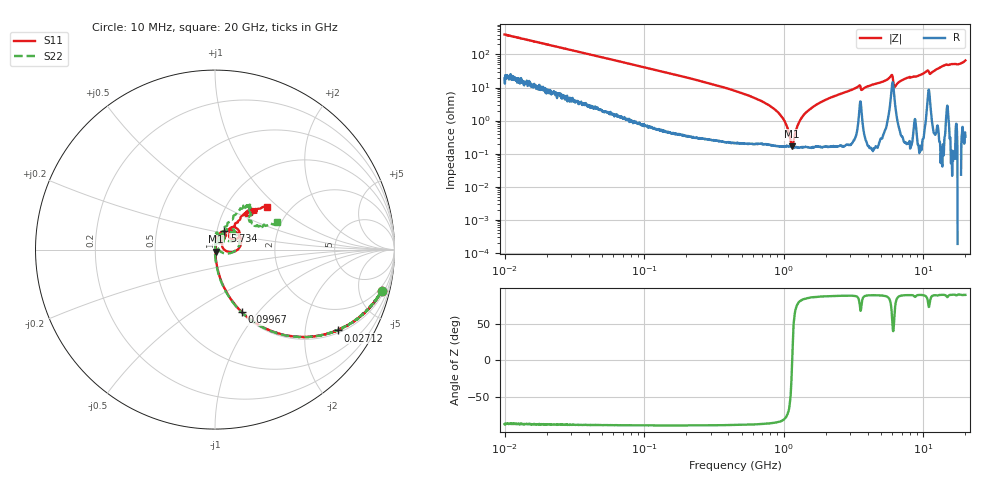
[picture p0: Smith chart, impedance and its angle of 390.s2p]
!Keysight Technologies,P5008B,MY61100088,A.16.20.02
!Date: Friday, August 30, 2024 14:09:02
!Correction: S11(C  2-Port  )
!S21(C  2-Port  )
!S12(C  2-Port  )
!S22(C  2-Port  )
!S2P File: Measurements: S11, S21, S12, S22:Log Frequency Sweep
# Hz S  MA  R 50
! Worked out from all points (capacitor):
!   1601 points, 10 MHz to 20 GHz, reference 50 ohm
!   read as one part in series: C = 39.7 pF near 10.39 MHz
!   lowest |Z| = 165 mohm at 1.146 GHz (marker M1)
!   series resonance near 1.147 GHz, so ESL is about 480 pH
!   S11 on the Smith chart (normalised r, x): 10 MHz: 1.36, -8.01; 27.12 MHz: 1.09, -2.97; 99.67 MHz: 1.01, -0.83; 5.734 GHz: 1.09, +0.23; 20 GHz: 1.53, +0.85
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1e7  0.9602 -13.8  0.2395 73.5  0.2395 73.5  0.9597 -13.9
2.711816e7  0.8189 -33.4  0.5504 54.9  0.5502 54.9  0.8188 -33.5
3.555162e7  0.7423 -40.4  0.6483 47.8  0.6482 47.8  0.7422 -40.5
9.966934e7  0.3793 -66.8  0.9191 22.1  0.9189 22.1  0.3794 -67.0
1.263918e8  0.3084 -71.2  0.9466 17.8  0.9462 17.8  0.3085 -71.4
4.472136e8  0.08415 -83.5  0.9945 4.2  0.9942 4.2  0.08405 -85.1
8.452326e8  0.03253 -83.5  0.9978 0.8  0.9975 0.8  0.03234 -89.0
1.145559e9  0.01272 -70.7  0.9984 -0.7  0.9982 -0.7  0.01214 -95.5
1.253768e9  0.007074 -60.9  0.9986 -1.1  0.9982 -1.1  0.00637 -96.4
1.378733e9  0.002306 0.7  0.9987 -1.6  0.9983 -1.6  0.000948 7.0
1.589917e9  0.00793 67.0  0.9987 -2.4  0.9983 -2.4  0.00716 84.9
2.114282e9  0.02432 80.2  0.9984 -4.1  0.9981 -4.1  0.0239 83.0
5.652411e9  0.1072 68.5  0.9805 -15.3  0.9803 -15.4  0.1088 63.1
5.733545e9  0.1168 63.4  0.9719 -16.0  0.9717 -16.0  0.116 60.7
5.927413e9  0.1531 40.2  0.9083 -16.9  0.9078 -17.0  0.146 33.8
6.425969e9  0.04667 30.1  0.9881 -12.4  0.9875 -12.5  0.03163 81.2
7.697294e9  0.09098 56.6  0.9973 -17.7  0.9969 -17.8  0.08744 82.3
9.08967e9  0.07903 57.0  0.9981 -21.4  0.9978 -21.4  0.07615 73.7
1.053187e10  0.1466 54.7  0.9774 -27.2  0.9774 -27.3  0.1365 54.5
1.141771e10  0.1189 46.8  0.9853 -26.1  0.9849 -26.2  0.1077 63.8
1.400536e10  0.2953 48.2  0.9666 -36.0  0.9663 -36.2  0.2901 56.8
2e10  0.3758 39.7  0.9293 -57.5  0.9288 -57.6  0.3793 23.9
